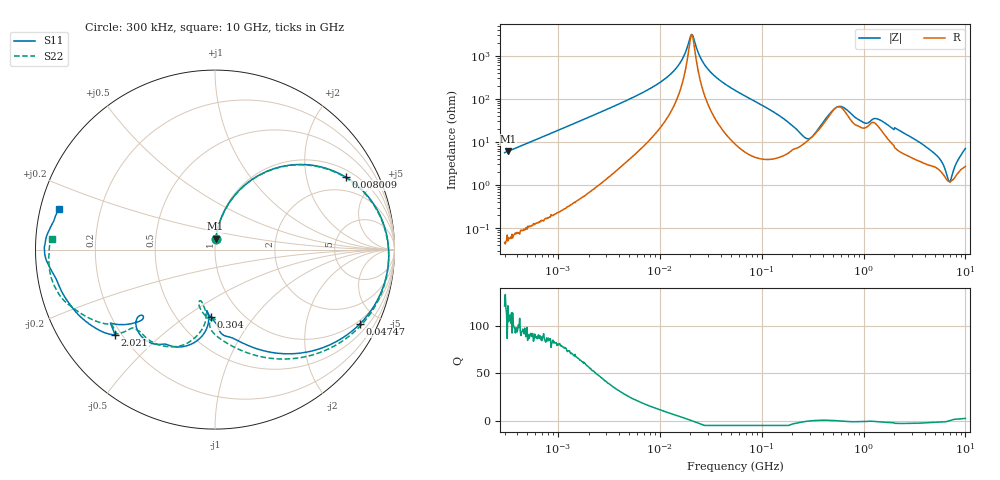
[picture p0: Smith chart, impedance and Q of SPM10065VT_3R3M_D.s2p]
! S-Parameter Data Generated by TDK Corporation
! Copyright(C) 2020 TDK Corporation.
! All Rights Reserved.
! TDK P/N: SPM10065VT-3R3M-D (Inductor)
! Property: L=3.3uH at 100kHz
! Size(LxWxT): 10.5x10x6.5mm
! Model Type: s2p (Touchstone File Format Version 1.0)
! Frequency: DC=Yes Start=0.3MHz Stop=10000MHz 802points Log-sweep
! Model Generated on Apr. 23, 2020
! Port Assignments:
!  1 ---@@@--- 2
! Applicable Conditions:
!  Temperature = 25 degC
!  DC Bias Current = 0 A
!  Small Signal Operation
! Terms and conditions regarding TDK Simulation Models
! (1)This simulation model is being provided solely for informational purposes. Please refer to the specifications of the products in terms of detailed characteristics of such products.
! (2)In no event shall TDK Corporation of any of its subsidiaries be liable for any loss or damage arising, directly or indirectly,
!  From any information contained in this simulation model, including, but not limited to loss or damages arising from any inaccuracies, omissions or errors in connection with such information.
! (3)Any and all copyrights on this simulation model are owned by TDK Corporation.
!  Duplication or redistribution of this simulation model without prior written permission from TDK Corporation is prohibited.
! (4)This simulation model is subject to any modification or change without any prior notice.
! (5)Neither TDK Corporation nor any of its subsidiaries shall make any warranty, express or implied,
!  Including but not limited to the correctness, implied warranties of merchantability and fitness for a particular purpose with respect to this simulation models.
! (6)The use of this simulation model shall be deemed to have consented to the terms and conditions hereof.
# Hz S MA R 50
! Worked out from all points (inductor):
!   801 points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, 300 kHz to 10 GHz, reference 50 ohm
!   read as 1/Y11, port 2 shorted: L = 2.97 uH near 318.3 kHz
!   highest Q = 113 at 322.9 kHz (marker M1), where L = 2.98 uH
!   self-resonance near 20.62 MHz
!   S11 on the Smith chart (normalised r, x): 300 kHz: 1.00, +0.11; 8.009 MHz: 1.29, +3.40; 47.47 MHz: 0.85, -3.95; 304 MHz: 0.72, -0.63; 2.021 GHz: 0.18, -0.36; 10 GHz: 0.05, +0.13
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300000  0.05679 87.1  0.9971 -3.2  0.9975 -3.2  0.05677 86.9
322921  0.06088 86.7  0.997 -3.4  0.9974 -3.5  0.06082 86.3
1713600  0.2991 71.5  0.9496 -17.7  0.9492 -17.7  0.2991 71.4
4239428  0.6145 49.6  0.7686 -38.6  0.7683 -38.6  0.6146 49.4
8009306  0.8323 29.1  0.5039 -57.5  0.5038 -57.5  0.8324 28.7
9671944  0.8784 23.0  0.4134 -62.7  0.4133 -62.7  0.8785 22.5
1.626666e7  0.9548 7.0  0.164 -72.2  0.164 -72.2  0.9549 6.3
2.28389e7  0.9691 -3.2  0.0305 -4.1  0.0305 -4.1  0.9692 -4.2
3.118733e7  0.9593 -12.9  0.151 65.3  0.151 65.3  0.9594 -14.3
4.746882e7  0.9067 -27.3  0.3539 57.0  0.3538 57.0  0.9067 -29.4
5.477226e7  0.8772 -32.6  0.4232 52.3  0.4231 52.3  0.8771 -35.1
8.974917e7  0.7325 -52.2  0.6408 32.5  0.6406 32.5  0.7314 -56.4
1.473106e8  0.5594 -71.6  0.7811 9.8  0.7808 9.8  0.5524 -79.0
3.040112e8  0.3759 -93.7  0.8154 -25.4  0.8152 -25.4  0.3551 -101.4
3.126428e8  0.3723 -94.2  0.8125 -27.0  0.8123 -27.0  0.3506 -102.1
5.225392e8  0.3618 -96.0  0.6569 -61.8  0.6567 -61.8  0.2998 -104.3
9.330971e8  0.6248 -122.6  0.378 -75.8  0.3779 -75.8  0.5825 -112.0
1.24442e9  0.5453 -137.5  0.399 -98.6  0.3989 -98.6  0.6195 -131.3
1.767019e9  0.6599 -140.7  0.2622 -141.4  0.262 -141.4  0.6674 -137.4
2.020878e9  0.7322 -139.4  0.2008 -156.5  0.2005 -156.4  0.7103 -144.0
5.21579e9  0.9039 -170.3  0.0197 161.1  0.01971 161.2  0.9124 -165.9
1e10  0.8992 165.3  0.01907 134.5  0.01904 135.0  0.9091 176.3
